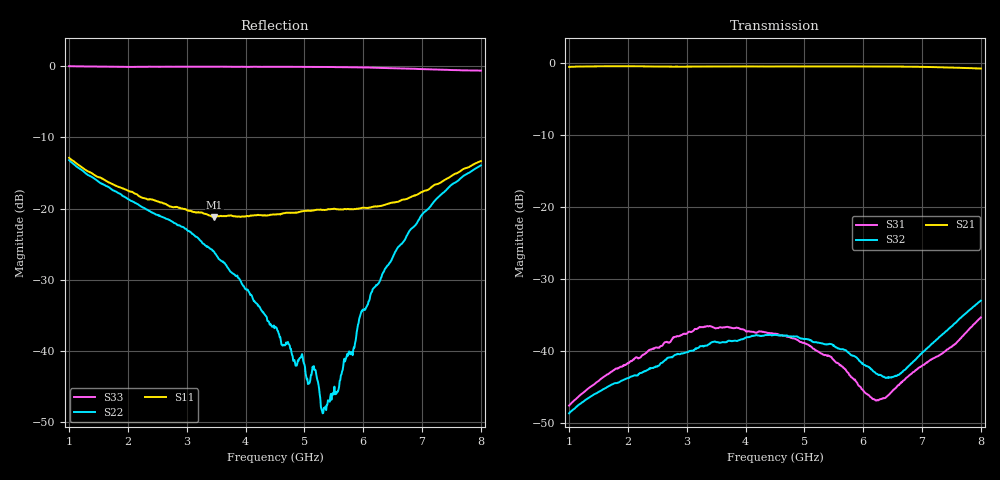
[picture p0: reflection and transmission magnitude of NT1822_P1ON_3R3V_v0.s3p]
! NT1822 PC-P1 ON state
! Port1:PC, Port2:P1, Port3:P2
! VDD=3.3V, VCTL=0V
# hz S ma R 50
! 3 Port Network Data from SP1.SP block
! freq  magS11  angS11  magS12  angS12  magS13  angS13
!  magS21  angS21
!  magS22  angS22  magS23  angS23
!  magS31  angS31  magS32  angS32
!  magS33  angS33
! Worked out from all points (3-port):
!   701 points, 1 GHz to 8 GHz, reference 50 ohm
!   strongest paths, dB at 1 GHz, 2.75 GHz, 4.5 GHz, 6.25 GHz, 8 GHz:
!     S21: -0.6, -0.6, -0.5, -0.5, -0.8
!     S32: -48.7, -40.9, -37.8, -43.3, -33.0
!     S31: -47.6, -38.4, -37.6, -46.9, -35.4
!   lowest |S11| = -21.2 dB at 3.47 GHz (marker M1), VSWR 1.19, Z = 54.3 - j8.06 ohm
!   |S11| at or under -10 dB: start of sweep to end of sweep
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1e9  0.2278 -77.4  0.936 1.5  0.004157 78.7
     0.9344 1.5  0.2194 -77.5  0.003688 73.6
     0.00416 78.8  0.003677 73.4  1.002 -12.4
3.47e9  0.0872 -57.6  0.9409 -30.3  0.01443 58.3
        0.94 -30.5  0.04929 -108.5  0.01157 66.8
        0.0144 57.8  0.01159 66.4  0.9943 -41.2
4.5e9  0.09092 -47.5  0.9414 -41.1  0.01318 46.3
       0.94 -41.2  0.0148 -170.5  0.0129 56.7
       0.01313 45.5  0.01286 56.3  0.9916 -53.7
4.97e9  0.09568 -52.3  0.9416 -45.9  0.01139 40.3
        0.9405 -46.0  0.009084 149.8  0.01209 51.7
        0.01134 39.7  0.01211 51.1  0.99 -60.5
5.06e9  0.09702 -53.3  0.9421 -46.9  0.01105 39.1
        0.941 -46.8  0.005854 138.1  0.01198 51.1
        0.01101 38.5  0.01196 50.4  0.9902 -61.9
5.17e9  0.09742 -55.1  0.9422 -48.0  0.01021 38.9
        0.9404 -47.8  0.007371 132.6  0.01144 51.1
        0.01026 38.0  0.01145 50.5  0.9881 -63.5
5.34e9  0.09771 -58.6  0.9425 -50.0  0.009338 40.2
        0.9413 -49.5  0.00398 130.7  0.0111 51.6
        0.009309 39.7  0.0111 50.4  0.9883 -66.3
6.24e9  0.104 -91.1  0.9411 -59.3  0.00456 76.7
        0.9395 -59.3  0.0292 -142.5  0.006898 66.0
        0.004557 75.9  0.006898 65.4  0.9768 -82.2
7.01e9  0.1316 -130.2  0.9349 -68.1  0.00792 120.9
        0.9342 -67.8  0.09183 -148.3  0.009725 115.1
        0.00792 119.8  0.009805 114.0  0.9559 -96.7
8e9  0.216 -169.0  0.9111 -79.0  0.01705 142.2
     0.9096 -79.1  0.2013 -149.4  0.02229 125.4
     0.01703 141.5  0.02228 124.8  0.9328 -112.6
